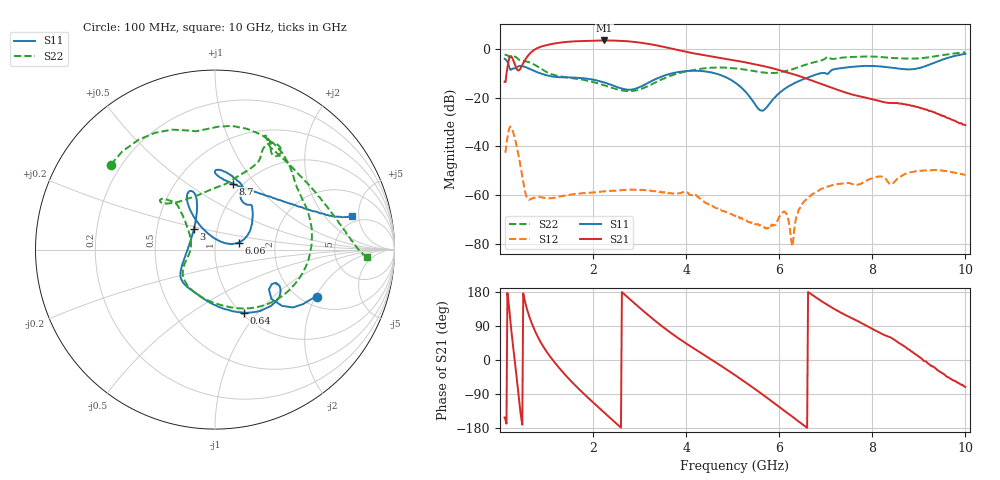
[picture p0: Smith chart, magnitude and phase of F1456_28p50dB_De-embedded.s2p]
! Integrated Device Technology
! Corporate Headquarters
! 6024 Silver Creek Valley Road
! San Jose, CA 95138  USA
! Phone:  1-408-284-8200
! Toll Free:  1-800-223-1366
! Webpage:  http://www.idt.com/
! Timing and RF Division
! 515 Groton Road, Suite 102
! Westford, MA 01886-6024
! Device:  F1456
! Description: 6-bit 0.5 dB Transmit Variable Gain Amplifier
! Frequency:  2100.0 -  2950.00 MHz
! Package:  6x6 mm Thin QFN Plastic Package: 28 pin
! State:  57
! Atten State:  28.5 dB
! Voltage:  +5.00 Volts
! Current:  216.933 mA
! Data:  The device was measured on a the F1455 evaluation board which has
!  individual transmission lines to the RF pins.  Data was collected
!  using a calibrated network analyzer.  The evaluation board was
!  de-embedded using a TRL calibration technique.
!  The reference plane is the edge of the package pin.
!  Pin  1 = CSb
!  Pin  2 = DATA
!  Pin  3 = CLK
!  Pin  4 = RSET
!  Pin  5 = GND
!  Pin  6 = RFIN  = Port 1
!  Pin  7 = GND
!  Pin  8 = NC
!  Pin  9 = NC
!  Pin 10 = NC
!  Pin 11 = NC
!  Pin 12 = NC
!  Pin 13 = NC
!  Pin 14 = /STBY
!  Pin 15 = GND
!  Pin 16 = RFOUT  = Port 2
!  Pin 17 = GND
!  Pin 18 = NC
!  Pin 19 = NC
!  Pin 20 = NC
!  Pin 21 = GND
!  Pin 22 = NC
!  Pin 23 = GND
!  Pin 24 = NC
!  Pin 25 = NC
!  Pin 26 = NC
!  Pin 27 = GND
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# GHz S dB R 50
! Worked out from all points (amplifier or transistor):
!   496 points, 100 MHz to 10 GHz, reference 50 ohm
!   highest |S21| = 3.4 dB at 2.24 GHz (marker M1)
!   |S21| within 3 dB of that: 819 MHz to 3.609 GHz (2.79 GHz wide, 126 % of centre)
!   unconditionally stable (mu >= 1): start of sweep to end of sweep
!   at 1.74 GHz: K = 282.89, MAG = 3.7 dB, |S12| = -59.3 dB
!   at 5.06 GHz: K = 1890.17, MAG = -3.9 dB, |S12| = -68.6 dB
!   at 10 GHz: K = 768.01, MAG = -21.7 dB, |S12| = -51.7 dB
!   S11 on the Smith chart (normalised r, x): 100 MHz: 2.37, -2.04; 640 MHz: 1.03, -0.85; 3 GHz: 0.77, +0.18; 6.06 GHz: 1.30, +0.10; 8.7 GHz: 0.90, +0.78; 10 GHz: 4.20, +4.14
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0.1  -4.10 -24.9  -13.55 -151.8  -42.28 50.4  -2.51 140.7
0.18  -6.24 -40.0  -5.52 157.9  -34.20 -2.5  -2.97 109.7
0.26  -8.26 -28.6  -3.64 59.6  -32.90 -100.4  -3.29 88.7
0.4  -7.16 -34.0  -8.94 -94.6  -43.73 150.2  -4.36 44.4
0.52  -7.34 -50.8  -5.25 163.9  -56.65 116.9  -5.07 21.0
0.64  -8.26 -65.5  -2.02 111.5  -61.79 140.2  -5.62 -6.2
0.82  -9.75 -84.0  0.40 59.4  -60.74 120.4  -7.44 -44.9
1.14  -11.43 -110.8  2.03 -1.0  -61.17 86.0  -10.62 -92.4
1.76  -12.04 -139.1  3.18 -84.3  -59.13 52.7  -12.64 -139.3
2.24  -13.82 -154.4  3.39 -138.7  -58.45 35.7  -14.97 -157.5
2.62  -16.33 179.9  3.22 179.3  -57.95 22.1  -17.10 -175.5
3  -15.70 136.4  2.53 137.9  -57.77 4.0  -16.70 157.4
3.4  -11.98 113.4  1.23 97.0  -58.42 -11.7  -13.29 138.1
4.14  -9.01 113.1  -1.81 32.6  -59.75 -44.9  -8.81 131.9
5.06  -13.94 122.9  -4.84 -40.7  -68.55 -90.9  -8.04 138.7
5.62  -25.35 66.5  -6.93 -89.1  -72.39 175.8  -9.65 124.3
6.06  -17.22 16.6  -9.09 -129.5  -67.38 140.0  -9.47 93.5
6.28  -14.55 22.0  -10.30 -149.3  -80.88 140.9  -8.46 79.4
6.7  -11.18 40.8  -13.01 172.5  -59.69 142.0  -5.80 65.2
8.36  -7.63 88.5  -22.19 61.4  -55.18 56.7  -3.70 62.4
8.7  -8.38 75.0  -22.76 34.9  -51.29 66.2  -4.01 51.2
10  -2.08 13.8  -31.31 -71.3  -51.71 -26.6  -1.46 -2.6
